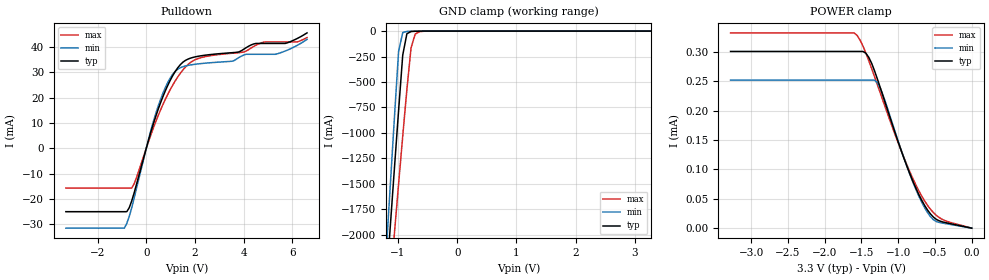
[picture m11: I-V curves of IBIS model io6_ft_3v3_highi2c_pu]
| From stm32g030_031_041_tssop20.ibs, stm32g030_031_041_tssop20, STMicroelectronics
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[Model]  io6_ft_3v3_highi2c_pu
Model_type I/O_open_drain
Polarity   Non-Inverting
Enable   Active-Low
Vinl =   0.990000V
Vinh =   2.310000V
Vmeas =  1.650000V
Cref =   50.000000pF
Rref =   100.000000M
Vref =   0.0V
C_comp   1.290400pF   1.272500pF   1.305600pF
[Temperature Range]   25.000000   -40.000000   0.125000k
[Pullup Reference]   3.300000V   3.000000V   3.600000V
[Pulldown Reference]   0.0V   0.0V   0.0V
[POWER Clamp Reference]   3.300000V   3.000000V   3.600000V
[GND Clamp Reference]   0.0V   0.0V   0.0V
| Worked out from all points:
|   slope of the pulldown table from 0 to 0.495 V, typ, clamps not added: 31.8 ohm
|   GND clamp passes 1 mA (typ) near -0.65 V on its own axis
[Pulldown]
|Voltage   I(typ)   I(min)   I(max)
-3.3V     -25.03mA   -31.54mA   -15.7mA
-900mV    -25.03mA   -31.54mA   -15.7mA
-700mV    -23.48mA   -26.95mA   -15.7mA
-500mV    -17.69mA   -19.75mA   -14.07mA
100mV     3.479mA    3.853mA    2.862mA
500mV     15.71mA    16.96mA    13.17mA
900mV     25.22mA    26.33mA    21.66mA
1.3V      31.91mA    31.32mA    28.29mA
2.2V      36.48mA    33.43mA    35.69mA
4.1V      39.76mA    37.15mA    38.42mA
5.3V      41.43mA    37.15mA    42.02mA
6.6V      45.6mA     43.04mA    43.74mA
[GND_clamp]
|Voltage   I(typ)   I(min)   I(max)
-3.3V     -9.61A     -9.635A    -9.699A
-1.2V     -2.493A    -2.184A    -2.958A
-1.13V    -1.917A    -1.512A    -2.469A
-1.06V    -1.345A    -845.6mA   -1.983A
-990mV    -779.8mA   -200.2mA   -1.503A
-920mV    -235.5mA   -14.18mA   -1.03A
-850mV    -26.06mA   -3.338mA   -574.2mA
-780mV    -4.499mA   -1.808mA   -166.4mA
-710mV    -1.722mA   -869.6uA   -29.45mA
-640mV    -806.7uA   -283.7uA   -6.281mA
3.28V     0A         0A         0A
[POWER_clamp]
|Voltage   I(typ)   I(min)   I(max)
-3.28V    300.8uA    252uA      332.4uA
-1.6V     300.8uA    252uA      332.4uA
-1.56V    300.8uA    252uA      328.4uA
-1.44V    297.9uA    252uA      298.3uA
-1.36V    280.4uA    252uA      271.4uA
-1.28V    252.9uA    246.9uA    243.1uA
-1.2V     222.5uA    224.3uA    214.5uA
-920mV    118.6uA    118.8uA    119.5uA
-680mV    47.6uA     44.33uA    54.63uA
-560mV    24.08uA    19.48uA    32.08uA
-480mV    14.89uA    11.29uA    21.67uA
0V        0A         0A         0A
[Ramp]
| variable   typ   min   max
dV/dt_r  1.07552/0.93429n   0.96306/0.90911n   1.029/1.06800n
dV/dt_f  1.03422/0.72440n   0.95490/0.75402n   1.02804/0.72299n
R_load = 50.000000
